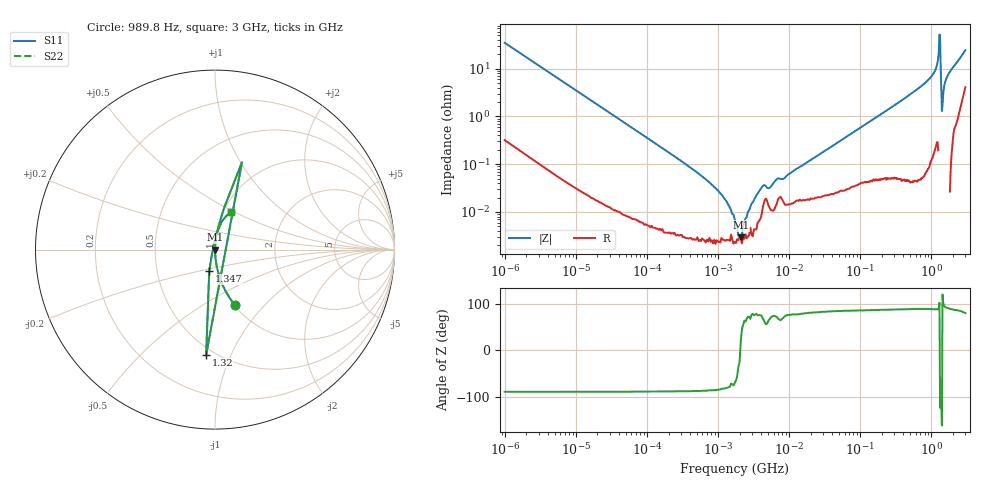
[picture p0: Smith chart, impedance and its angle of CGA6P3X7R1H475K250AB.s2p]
! S-Parameter Data Generated by TDK Corporation
! Copyright(C) 2020 TDK Corporation.
! All Rights Reserved.
! TDK P/N: CGA6P3X7R1H475K250AB (Multilayer Ceramic Chip Capacitor)
! Property: C=4.7uF
! Size(LxWxT): 3.2x2.5x2.5mm
! Model Type: s2p (Touchstone File Format Version 1.0)
! Frequency: DC=Yes Start=0.000989846MHz Stop=3000MHz 463points Log-sweep
! Model Generated on Aug. 18, 2020
! Port Assignments:
!  1 ---| |--- 2
! Applicable Conditions:
!  Temperature = 25 degC
!  DC Bias Voltage = 0 V
!  Small Signal Operation
! Terms and conditions regarding TDK Simulation Models
! (1)This simulation model is being provided solely for informational purposes. Please refer to the specifications of the products in terms of detailed characteristics of such products.
! (2)In no event shall TDK Corporation of any of its subsidiaries be liable for any loss or damage arising, directly or indirectly,
!  From any information contained in this simulation model, including, but not limited to loss or damages arising from any inaccuracies, omissions or errors in connection with such information.
! (3)Any and all copyrights on this simulation model are owned by TDK Corporation.
!  Duplication or redistribution of this simulation model without prior written permission from TDK Corporation is prohibited.
! (4)This simulation model is subject to any modification or change without any prior notice.
! (5)Neither TDK Corporation nor any of its subsidiaries shall make any warranty, express or implied,
!  Including but not limited to the correctness, implied warranties of merchantability and fitness for a particular purpose with respect to this simulation models.
! (6)The use of this simulation model shall be deemed to have consented to the terms and conditions hereof.
# Hz S MA R 50
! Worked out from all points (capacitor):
!   462 points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, 989.8 Hz to 3 GHz, reference 50 ohm
!   read as one part in series: C = 4.59 uF near 1.07 kHz
!   lowest |Z| = 2.93 mohm at 2.074 MHz (marker M1)
!   series resonance near 2.045 MHz, so ESL is about 1.3 nH
!   S11 on the Smith chart (normalised r, x): 989.8 Hz: 1.01, -0.70; 1.32 GHz: 0.45, -0.81; 1.347 GHz: 0.91, -0.22; 3 GHz: 1.08, +0.48
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989.846  0.3288 -70.3  0.9414 19.2  0.9414 19.2  0.3288 -70.3
12024.64  0.02934 -87.8  0.9993 1.7  0.9993 1.7  0.02934 -87.8
146075.1  0.002443 -88.9  1 0.1  1 0.1  0.002443 -88.9
695650.9  0.0004603 -86.7  1 0.0  1 0.0  0.0004603 -86.7
1774518  5.402e-05 -65.5  1 0.0  1 0.0  5.402e-05 -65.5
2074254  2.934e-05 16.8  1 -0.0  1 -0.0  2.934e-05 16.8
2621405  0.0001023 72.6  1 -0.0  1 -0.0  0.0001023 72.6
4186766  0.0003459 70.8  0.9999 -0.0  0.9999 -0.0  0.0003459 70.8
2.073191e7  0.001268 81.4  0.9998 -0.1  0.9998 -0.1  0.001268 81.4
2.507343e8  0.01426 87.2  0.9994 -0.8  0.9994 -0.8  0.01426 87.2
9.395906e8  0.06186 85.6  0.9972 -3.5  0.9972 -3.5  0.06186 85.6
1.147801e9  0.09759 83.1  0.993 -5.6  0.993 -5.6  0.09759 83.1
1.243477e9  0.1651 79.8  0.9844 -9.5  0.9844 -9.5  0.1651 79.8
1.268618e9  0.2311 77.9  0.9781 -13.4  0.9781 -13.4  0.2311 77.9
1.320433e9  0.587 -94.8  1.201 29.1  1.201 29.1  0.587 -94.8
1.347129e9  0.122 -105.2  1.039 6.5  1.039 6.5  0.122 -105.2
1.374365e9  0.04238 -116.5  1.02 2.1  1.02 2.1  0.04238 -116.5
1.402151e9  0.01318 -161.9  1.013 0.2  1.013 0.2  0.01318 -161.9
1.45942e9  0.02869 102.0  1.006 -1.6  1.006 -1.6  0.02869 102.0
1.54974e9  0.0513 91.0  1.002 -2.9  1.002 -2.9  0.0513 91.0
1.67892e9  0.07044 87.2  0.999 -4.0  0.999 -4.0  0.07044 87.2
3e9  0.2295 67.3  0.9357 -13.1  0.9357 -13.1  0.2295 67.3
